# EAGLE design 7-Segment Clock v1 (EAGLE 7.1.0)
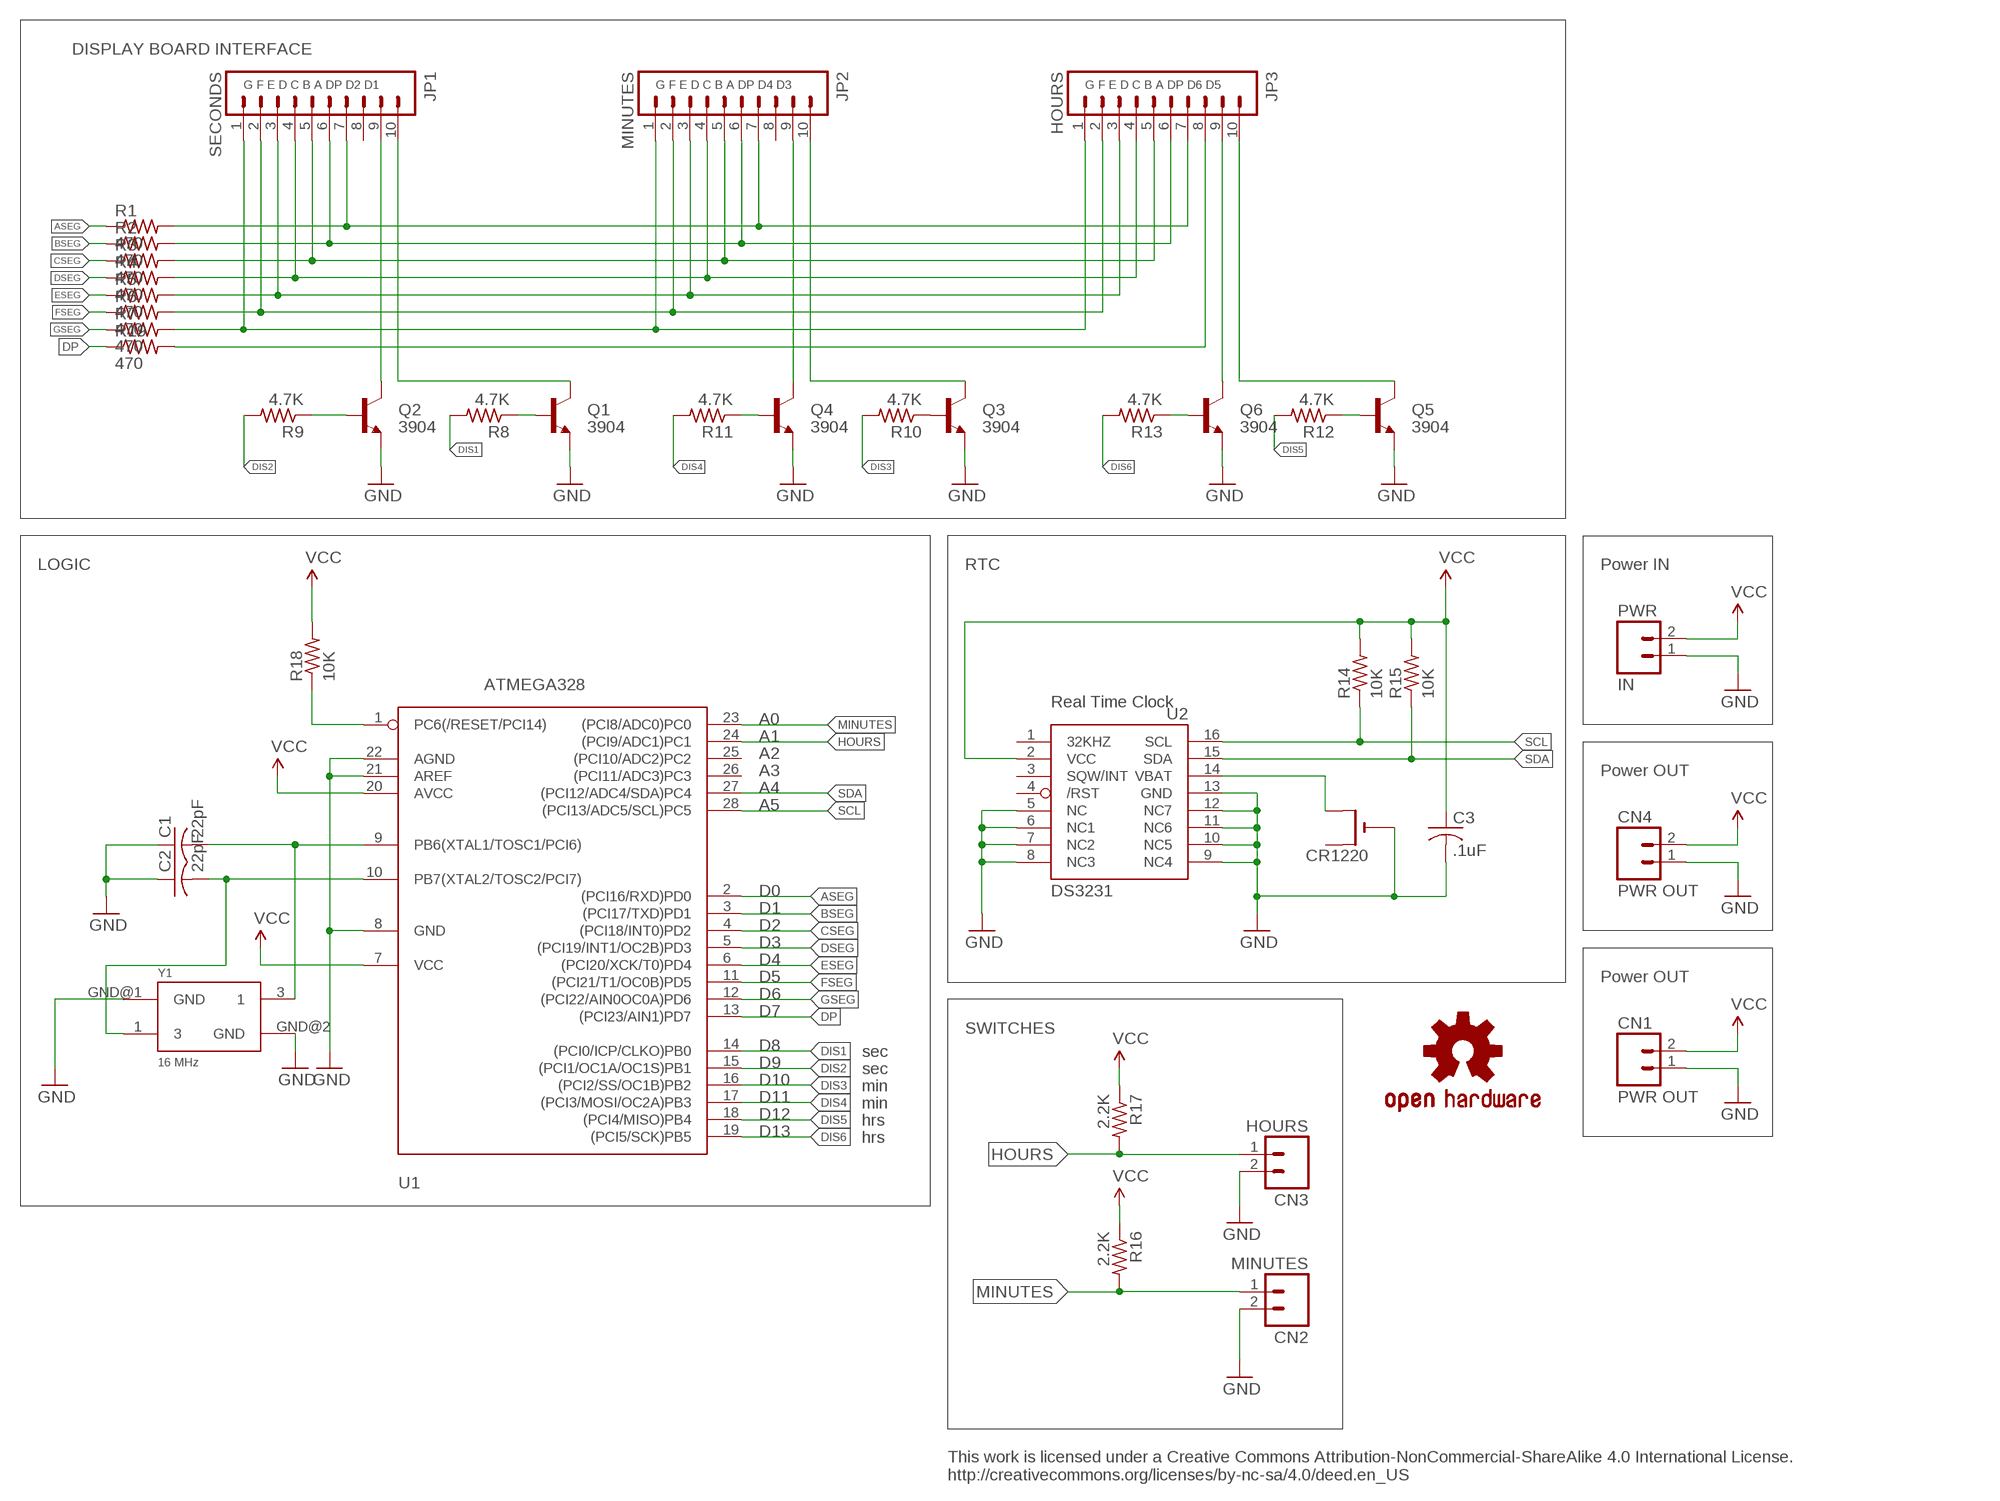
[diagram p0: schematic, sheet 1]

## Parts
C1  22pF  C-USC0805K  [C0805K]
C2  22pF  C-USC0805K  [C0805K]
C3  .1uF  C-USC0805K  [C0805K]
CN1  PWR OUT  M02PTH  [1X02]
CN2  MINUTES  M02PTH  [1X02]
CN3  HOURS  M02PTH  [1X02]
CN4  PWR OUT  M02PTH  [1X02]
CR1220  CR1220THM  [CR1220-THM]
JP1  SECONDS  M10NO_SILK  [1X10_NO_SILK]
JP2  MINUTES  M10NO_SILK  [1X10_NO_SILK]
JP3  HOURS  M10NO_SILK  [1X10_NO_SILK]
PWR  IN  M02PTH  [1X02]
Q1  3904  TRANSISTOR_NPNMMBT2222A  [SOT23]
Q2  3904  TRANSISTOR_NPNMMBT2222A  [SOT23]
Q3  3904  TRANSISTOR_NPNMMBT2222A  [SOT23]
Q4  3904  TRANSISTOR_NPNMMBT2222A  [SOT23]
Q5  3904  TRANSISTOR_NPNMMBT2222A  [SOT23]
Q6  3904  TRANSISTOR_NPNMMBT2222A  [SOT23]
R1  470  R-US_R0805  [R0805]
R2  470  R-US_R0805  [R0805]
R3  470  R-US_R0805  [R0805]
R4  470  R-US_R0805  [R0805]
R5  470  R-US_R0805  [R0805]
R6  470  R-US_R0805  [R0805]
R7  470  R-US_R0805  [R0805]
R8  4.7K  R-US_R0805  [R0805]
R9  4.7K  R-US_R0805  [R0805]
R10  4.7K  R-US_R0805  [R0805]
R11  4.7K  R-US_R0805  [R0805]
R12  4.7K  R-US_R0805  [R0805]
R13  4.7K  R-US_R0805  [R0805]
R14  10K  R-US_R0805  [R0805]
R15  10K  R-US_R0805  [R0805]
R16  2.2K  R-US_R0805  [R0805]
R17  2.2K  R-US_R0805  [R0805]
R18  10K  R-US_R0805  [R0805]
R19  470  R-US_R0805  [R0805]
U1  ATMEGA328  ATMEGA168PROUND  [DIL28-3-ROUND]
U2  DS3231  DS3231/SO  [SO16W]
U$7  OSHW-LOGOS  [OSHW-LOGO-S]
Y1  16 MHz  OSCILLATOR5X3  [CRYSTAL-SMD-5X3]

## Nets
ASEG: R1.1 U1.2((PCI16/RXD)PD0)
BSEG: R2.1 U1.3((PCI17/TXD)PD1)
CSEG: R3.1 U1.4((PCI18/INT0)PD2)
DIS1: R8.2 U1.14((PCI0/ICP/CLKO)PB0)
DIS2: R9.2 U1.15((PCI1/OC1A/OC1S)PB1)
DIS3: R10.2 U1.16((PCI2/SS/OC1B)PB2)
DIS4: R11.2 U1.17((PCI3/MOSI/OC2A)PB3)
DIS5: R12.2 U1.18((PCI4/MISO)PB4)
DIS6: R13.2 U1.19((PCI5/SCK)PB5)
DP: R19.1 U1.13((PCI23/AIN1)PD7)
DSEG: R4.1 U1.5((PCI19/INT1/OC2B)PD3)
ESEG: R5.1 U1.6((PCI20/XCK/T0)PD4)
FSEG: R6.1 U1.11((PCI21/T1/OC0B)PD5)
GND: C1.1 C2.1 C3.2 CN1.1 CN2.2 CN3.2 CN4.1 CR1220.- PWR.1 Q1.2(E) Q2.2(E) Q3.2(E) Q4.2(E) Q5.2(E) Q6.2(E) U1.8(GND) U1.21(AREF) U1.22(AGND) U2.5(NC) U2.6(NC1) U2.7(NC2) U2.8(NC3) U2.9(NC4) U2.10(NC5) U2.11(NC6) U2.12(NC7) U2.13(GND) Y1.GND@1(GND) Y1.GND@2(GND)
GSEG: R7.1 U1.12((PCI22/AIN0OC0A)PD6)
HOURS: CN3.1 R17.2 U1.24((PCI9/ADC1)PC1)
MINUTES: CN2.1 R16.2 U1.23((PCI8/ADC0)PC0)
N$1: Q1.1(B) R8.1
N$2: CR1220.+2(+1) U2.14(VBAT)
N$3: Q2.1(B) R9.1
N$4: JP1.7 JP2.7 JP3.7 R1.2
N$5: JP1.6 JP2.6 JP3.6 R2.2
N$6: JP1.5 JP2.5 JP3.5 R3.2
N$7: JP1.4 JP2.4 JP3.4 R4.2
N$8: Q3.1(B) R10.1
N$9: JP1.2 JP2.2 JP3.2 R6.2
N$10: JP1.1 JP2.1 JP3.1 R7.2
N$11: JP3.8 R19.2
N$12: JP1.9 Q2.3(C)
N$13: JP1.10 Q1.3(C)
N$14: JP2.9 Q4.3(C)
N$15: Q4.1(B) R11.1
N$16: Q5.1(B) R12.1
N$17: Q6.1(B) R13.1
N$18: JP2.10 Q3.3(C)
N$19: JP3.9 Q6.3(C)
N$20: JP3.10 Q5.3(C)
N$24: JP1.3 JP2.3 JP3.3 R5.2
N$36: R18.1 U1.1(PC6(/RESET/PCI14))
N$37: C1.2 U1.9(PB6(XTAL1/TOSC1/PCI6)) Y1.3
N$38: C2.2 U1.10(PB7(XTAL2/TOSC2/PCI7)) Y1.1
SCL: R14.1 U1.28((PCI13/ADC5/SCL)PC5) U2.16(SCL)
SDA: R15.1 U1.27((PCI12/ADC4/SDA)PC4) U2.15(SDA)
VCC: C3.1 CN1.2 CN4.2 PWR.2 R14.2 R15.2 R16.1 R17.1 R18.2 U1.7(VCC) U1.20(AVCC) U2.2(VCC)
Unconnected: CR1220.+1(+) JP1.8 JP2.8 U1.25((PCI10/ADC2)PC2) U1.26((PCI11/ADC3)PC3) U2.1(32KHZ) U2.3(SQW/INT) U2.4(/RST)

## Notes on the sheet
- DISPLAY BOARD INTERFACE
- G F E D C B A DP D2 D1 | G F E D C B A DP D4 D3 | G F E D C B A DP D6 D5
- LOGIC | RTC | Power IN
- Real Time Clock
- A0
- A1
- A2
- A3 | Power OUT
- A4
- A5
- D0
- D1
- D2
- D3
- D4
- D5 | Power OUT
- D6
- D7
- SWITCHES
- D8 | sec
- D9 | sec
- D10 | min
- D11 | min
- D12 | hrs
- D13 | hrs
- This work is licensed under a Creative Commons Attribution-NonCommercial-ShareAlike 4.0 International License.
  http://creativecommons.org/licenses/by-nc-sa/4.0/deed.en_US

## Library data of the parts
C1-C3 = adafruit:C-US: CAPACITOR, American symbol
CN1-CN4 PWR = SparkFun w:epaper:M02: Header 2
CR1220 = adafruit:CR1220: CR1216/CR1220/CR1225 12mm 3V lithium coin cell Great for battery packup. Both SMT and THM holders. Note the THM package has the ground pads on both sides of the PCB so that the masks are the same - this reduces the cost
JP1-JP3 = SparkFun-Connectors:M10: Header 10 Standard 10-pin 0.1" header. Use with straight break away headers (SKU : PRT-00116), right angle break away headers (PRT-00553), swiss pins (PRT-00743), machine pins (PRT-00117), and female headers (PRT-00115).
Q1-Q6 = SparkFun-DiscreteSemi:TRANSISTOR_NPN: Generic NPN BJT MMBT2222A - TRANS-08049 (SOT-23, 1A 40V) MPSA42 - TRANS-09116 (SOT-23, 500mA 300V) MMBT5088LT1G - TRANS-11160 (SOT-23, 50 mA 30V); PROD_ID: TRANS-08049; VALUE: MMBT2222A
R1-R19 = adafruit:R-US_: RESISTOR, American symbol
U1 = adafruit:ATMEGA168*P: MICROCONTROLLER 16 kBytes FLASH 1 kBytes SRAM 512 Bytes EEPROM USART 8-channel 10 bit ADC
U2 = adafruit:DS3231
U$7 = SparkFun:OSHW-LOGO: Open Source Hardware Logo This logo indicates the piece of hardware it is found on incorporates a OSHW license and/or adheres to the definition of open source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
Y1 = SparkFun-FreqCtrl:OSCILLATOR: Generic 5x3 and 7x5 oscillators

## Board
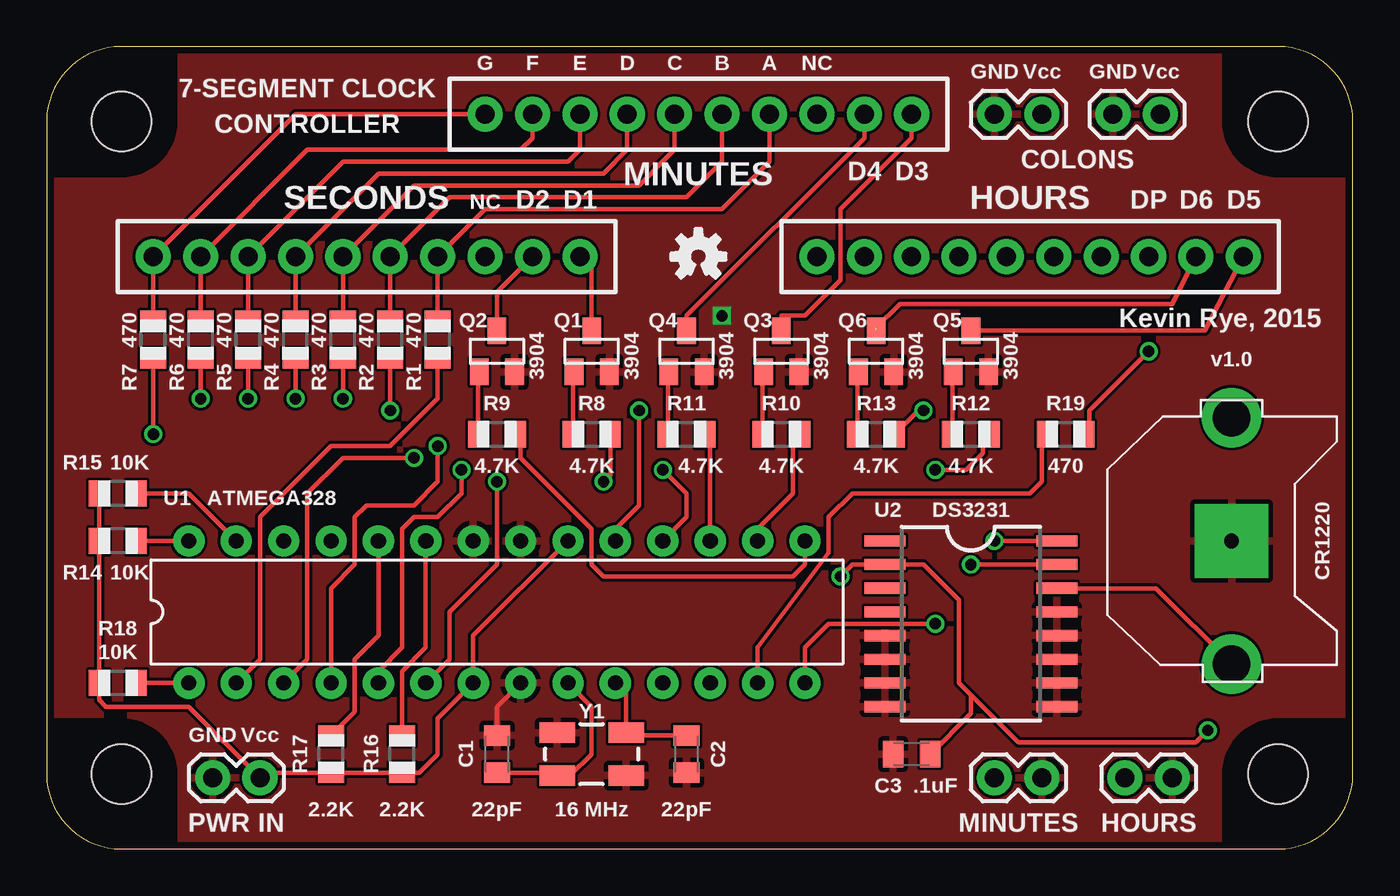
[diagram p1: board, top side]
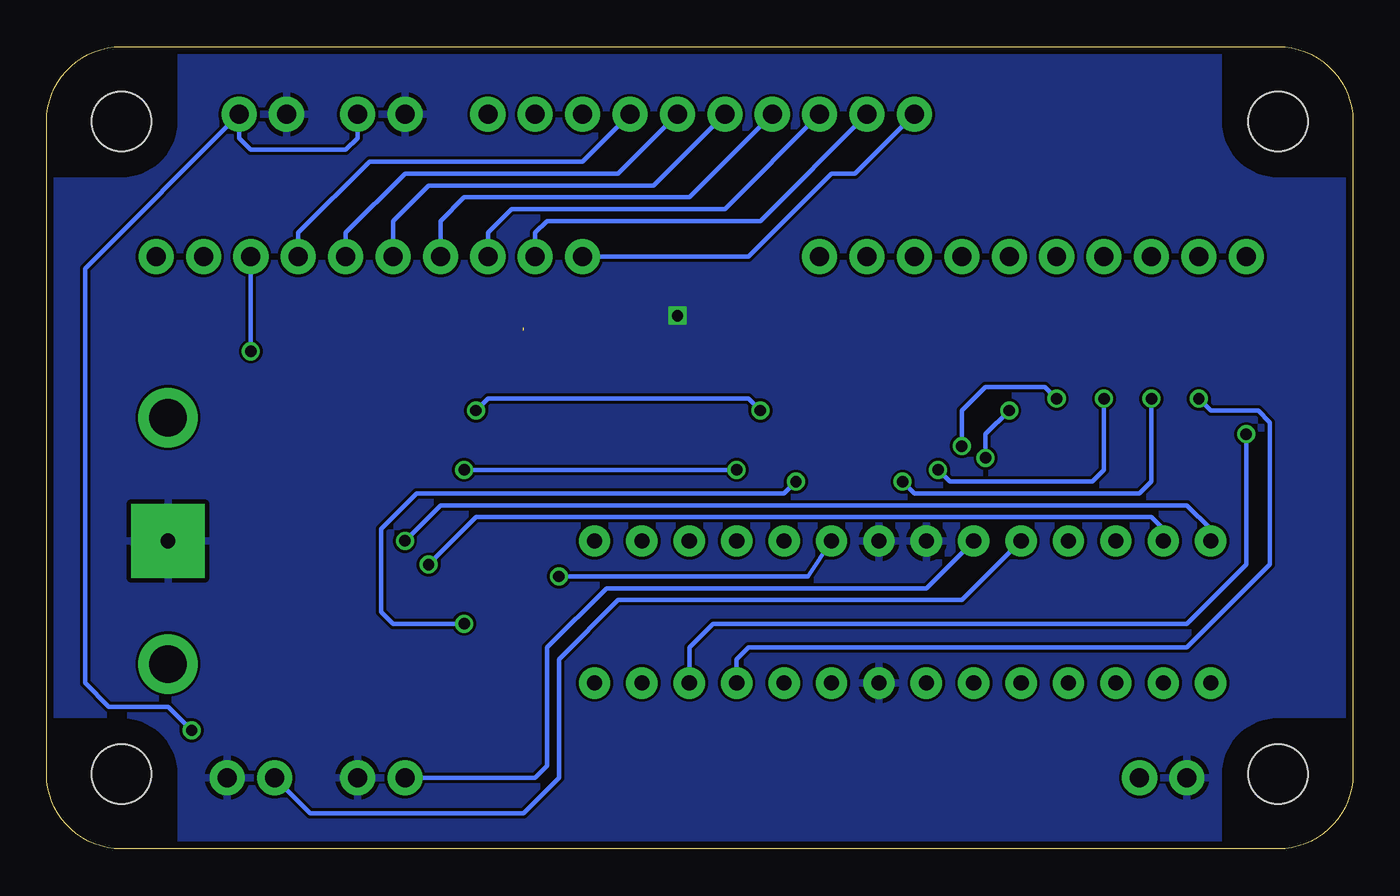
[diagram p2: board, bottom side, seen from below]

Size 70 x 43 mm. Coordinates in mm from the lower left corner, seen from the top.
Copper layers (1*16): Top 0.0356mm / dielectric 1.5011mm / Bottom 0.0356mm
Design rules "LaenPCBOrder": minimum track width 6mil, minimum drill 13mil, track to track 6mil, track to pad 6mil, pad to pad 6mil, via to via 6mil, smd to smd 6mil, copper to edge 15mil, drill to drill 6mil, minimum pad ring 7mil, minimum via ring 7mil, stop-mask expansion 3mil, vias tented up to drill 0mil, thermal gap 10mil

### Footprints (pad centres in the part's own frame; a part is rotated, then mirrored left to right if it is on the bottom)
C0805K = smd 1.1 x 1.4: 1 -1,0; 2 1,0
1X02 = drill 1.016 pad 1.88: 1 0,0; 2 2.54,0
CR1220-THM = drill 2 pad 3.175: +1 -6.604,0; +2 6.604,0 | drill 0.8 pad 3.962 square: - 0,0
1X10_NO_SILK = drill 1.016 pad 1.88: 1 0,0; 2 2.54,0; 3 5.08,0; 4 7.62,0; 5 10.16,0; 6 12.7,0; 7 15.24,0; 8 17.78,0; 9 20.32,0; 10 22.86,0
SOT23 = smd 1 x 1.4: 1 -0.95,-1.1; 2 0.95,-1.1; 3 0,1.1
R0805 = smd 1.1 x 1.4: 1 -1,0; 2 1,0
DIL28-3-ROUND = drill 0.813 pad 1.676: 1 -16.51,-3.81; 2 -13.97,-3.81; 3 -11.43,-3.81; 4 -8.89,-3.81; 5 -6.35,-3.81; 6 -3.81,-3.81; 7 -1.27,-3.81; 8 1.27,-3.81; 9 3.81,-3.81; 10 6.35,-3.81; 11 8.89,-3.81; 12 11.43,-3.81; 13 13.97,-3.81; 14 16.51,-3.81; 15 16.51,3.81; 16 13.97,3.81; 17 11.43,3.81; 18 8.89,3.81; 19 6.35,3.81; 20 3.81,3.81; 21 1.27,3.81; 22 -1.27,3.81; 23 -3.81,3.81; 24 -6.35,3.81; 25 -8.89,3.81; 26 -11.43,3.81; 27 -13.97,3.81; 28 -16.51,3.81
SO16W = smd 0.6 x 2.2: 1 -4.445,-4.6; 2 -3.175,-4.6; 3 -1.905,-4.6; 4 -0.635,-4.6; 5 0.635,-4.6; 6 1.905,-4.6; 7 3.175,-4.6; 8 4.445,-4.6; 9 4.445,4.6; 10 3.175,4.6; 11 1.905,4.6; 12 0.635,4.6; 13 -0.635,4.6; 14 -1.905,4.6; 15 -3.175,4.6; 16 -4.445,4.6
DP7043_V1 = hole 3.2: 4,4; 66,4; 66,39; 4,39
CRYSTAL-SMD-5X3 = smd 1.9 x 1.1: 1 -1.85,-1.15; 3 1.85,1.15; GND@1 -1.85,1.15; GND@2 1.85,-1.15

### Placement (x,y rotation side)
C1  24.13,5.08 270 top
C2  34.29,5.08 90 top
C3  46.35,5.08 180 top
CN1  50.8,39.37 0 top
CN2  50.8,3.81 0 top
CN3  57.78,3.81 0 top
CN4  57.15,39.37 0 top
CR1220  63.5,16.51 270 top
JP1  5.71,31.75 0 top
JP2  23.5,39.37 0 top
JP3  41.27,31.75 0 top
PWR  8.89,3.81 0 top
Q1  29.21,26.67 0 top
Q2  24.13,26.67 0 top
Q3  39.37,26.67 0 top
Q4  34.29,26.67 0 top
Q5  49.53,26.67 0 top
Q6  44.45,26.67 0 top
R1  20.95,27.31 90 top
R2  18.41,27.31 90 top
R3  15.88,27.31 90 top
R4  13.34,27.31 90 top
R5  10.79,27.31 90 top
R6  8.26,27.31 90 top
R7  5.71,27.31 90 top
R8  29.21,22.22 0 top
R9  24.13,22.22 0 top
R10  39.37,22.22 0 top
R11  34.29,22.22 0 top
R12  49.53,22.22 0 top
R13  44.45,22.22 0 top
R14  3.81,16.51 180 top
R15  3.81,19.05 180 top
R16  19.05,5.08 90 top
R17  15.24,5.08 90 top
R18  3.81,8.89 180 top
R19  54.61,22.22 0 top
U1  24.13,12.7 0 top
U2  49.53,12.07 270 top
U$2  [DP7043_V1]  0,0 0 top
U$7  34.92,31.75 0 top
Y1  29.21,5.08 180 top

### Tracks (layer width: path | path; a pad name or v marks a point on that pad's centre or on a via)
ASEG
  Top 0.254: U1.2 11.43,10.16 11.43,17.78 15.24,21.59 18.41,21.59 20.95,24.13 R1.1 20.95,24.77
BSEG  (via drill 0.61)
  Top 0.254: U1.3 13.97,10.16 13.97,19.05 15.88,20.96 v19.68,20.96 | v18.41,23.5 R2.1
  Bottom 0.254: v19.68,20.96 19.68,22.22 v18.41,23.5
CSEG  (via drill 0.61)
  Top 0.254: U1.4 15.24,13.97 16.51,15.24 16.51,17.78 17.14,18.41 19.68,18.41 20.95,19.68 v20.95,21.59 | v15.88,24.13 R3.1
  Bottom 0.254: v20.95,21.59 20.95,23.5 19.68,24.77 16.51,24.77 v15.88,24.13
DIS1  (via drill 0.61)
  Top 0.254: R8.2 30.21,20.05 v29.84,19.68 | v47.62,12.07 41.91,12.07 40.64,10.8 U1.14
  Bottom 0.254: v29.84,19.68 30.48,19.05 50.16,19.05 52.07,17.14 52.07,12.7 51.44,12.07 v47.62,12.07
DIS2
  Top 0.254: U1.15 40.64,15.24 40.01,14.61 29.84,14.61 29.21,15.24 29.21,17.14 25.4,20.96 25.4,21.96 R9.2
DIS3
  Top 0.254: U1.16 38.1,17.14 40.01,19.05 40.01,21.86 R10.2
DIS4
  Top 0.254: U1.17 35.56,21.96 R11.2
DIS5  (via drill 0.61)
  Top 0.254: v47.62,20.32 49.27,20.32 50.16,21.22 50.16,21.86 R12.2 | v33.02,20.32 34.29,19.05 34.29,17.78 U1.18
  Bottom 0.254: v33.02,20.32 v47.62,20.32
DIS6  (via drill 0.61)
  Top 0.254: U1.19 30.48,17.14 31.75,18.41 v31.75,23.5 | v46.99,23.5 46.72,23.5 R13.2
  Bottom 0.254: v31.75,23.5 32.38,24.13 46.35,24.13 v46.99,23.5
DP
  Top 0.254: U1.13 38.1,10.8 41.91,15.88 41.91,17.78 43.18,19.05 52.7,19.05 53.34,19.68 53.34,21.96 R19.1
DSEG  (via drill 0.61)
  Top 0.254: U1.5 17.78,9.53 19.05,10.8 19.05,17.14 19.68,17.78 20.95,17.78 22.23,19.05 v22.23,20.32 | R4.1 v13.34,24.13
  Bottom 0.254: v13.34,24.13 13.34,20.32 13.97,19.68 21.59,19.68 v22.23,20.32
ESEG  (via drill 0.61)
  Top 0.254: U1.6 21.59,10.16 21.59,12.7 24.13,15.24 v24.13,19.68 | v10.79,24.13 R5.1
  Bottom 0.254: v24.13,19.68 23.5,19.05 11.43,19.05 10.79,19.68 v10.79,24.13
FSEG  (via drill 0.61)
  Top 0.254: v8.26,24.13 R6.1
  Bottom 0.254: U1.11 33.02,10.16 32.38,10.8 8.89,10.8 4.45,15.24 4.45,22.86 5.08,23.5 7.62,23.5 v8.26,24.13
GND  (via drill 0.61)
  Top 0.254: C1.1 24.13,7.62 U1.8
  other vias: 36.2,28.57
  pour Top: -1.27,44.45 71.75,44.45 71.75,-1.27 -1.27,-1.27
  pour Bottom: -0.64,43.81 71.12,43.81 71.12,-0.63 -0.64,-0.63
GSEG  (via drill 0.61)
  Top 0.254: v5.71,22.22 R7.1
  Bottom 0.254: U1.12 35.56,10.8 34.29,12.07 8.89,12.07 5.71,15.24 v5.71,22.22
HOURS
  Top 0.254: 15.24,6.35 R17.2 16.51,7.35 16.51,10.16 17.78,11.43 U1.24
  Bottom 0.254: CN3.1 55.88,1.91 44.45,1.91 42.55,3.81 42.55,10.16 39.37,13.34 20.95,13.34 U1.24
MINUTES
  Top 0.254: R16.2 19.05,9.53 20.32,10.8 U1.23
  Bottom 0.254: CN2.1 43.81,3.81 43.18,4.45 43.18,10.8 40.01,13.97 22.86,13.97 U1.23
N$1
  Top 0.254: R8.1 28.21,25.52 Q1.1
N$2
  Top 0.254: U2.14 59.44,13.97 CR1220.+2
N$3
  Top 0.254: R9.1 23.13,25.52 Q2.1
N$4
  Top 0.254: R1.2 JP1.7 23.5,34.29 36.2,34.29 38.73,36.83 JP2.7
  Bottom 0.254: JP3.7 56.52,33.02 52.7,36.83 41.27,36.83 JP2.7
N$5
  Top 0.254: R2.2 JP1.6 21.59,34.92 34.29,34.92 36.2,36.83 JP2.6
  Bottom 0.254: JP3.6 53.98,33.02 50.8,36.2 39.37,36.2 JP2.6
N$6
  Top 0.254: R3.2 JP1.5 19.68,35.56 31.75,35.56 33.66,37.47 JP2.5
  Bottom 0.254: JP2.5 37.47,35.56 49.53,35.56 51.44,33.66 JP3.5
N$7
  Top 0.254: R4.2 JP1.4 17.78,36.2 29.84,36.2 31.11,37.47 JP2.4
  Bottom 0.254: JP3.4 48.9,33.66 47.62,34.92 35.56,34.92 JP2.4
N$8
  Top 0.254: R10.1 38.37,25.52 Q3.1
N$9
  Top 0.254: R6.2 JP1.2 13.97,37.47 25.4,37.47 26.04,38.1 JP2.2
  Bottom 0.254: JP3.2 43.81,33.02 43.18,33.66 31.75,33.66 JP2.2
N$10
  Top 0.254: R7.2 JP1.1 13.34,39.37 JP2.1
  Bottom 0.254: JP3.1 32.38,31.75 27.94,36.2 26.67,36.2 JP2.1
N$11  (via drill 0.61)
  Top 0.254: v59.05,26.67 55.88,23.5 55.88,22.5 R19.2
  Bottom 0.254: v59.05,26.67 JP3.8
N$12
  Top 0.254: Q2.3 24.13,29.85 JP1.9
N$13
  Top 0.254: Q1.3 29.21,31.11 JP1.10
N$14
  Top 0.254: Q4.3 34.29,28.57 43.81,38.1 JP2.9
N$15
  Top 0.254: R11.1 33.29,25.52 Q4.1
N$16
  Top 0.254: R12.1 48.53,25.52 Q5.1
N$17
  Top 0.254: R13.1 43.45,25.52 Q6.1
N$18
  Top 0.254: Q3.3 39.37,28.57 40.64,28.57 42.55,30.48 42.55,34.29 46.35,38.1 JP2.10
N$19  (1 unrouted)
  Top 0.254: 44.45,27.94 45.72,29.21 60.33,29.21 JP3.9
N$20
  Top 0.254: Q5.3 62.06,27.77 JP3.10
N$24
  Top 0.254: R5.2 JP1.3 15.88,36.83 27.94,36.83 28.57,37.47 JP2.3
  Bottom 0.254: JP3.3 46.35,33.02 45.09,34.29 33.66,34.29 JP2.3
N$36
  Top 0.254: R18.1 U1.1
N$37
  Top 0.254: U1.9 29.21,7.62 29.21,5.08 28.06,3.93 Y1.3 27.21,4.08 C1.2
N$38
  Top 0.254: U1.10 31.06,8.31 Y1.1 31.21,6.08 C2.2
SCL  (via drill 0.61)
  Top 0.254: v50.8,16.51 U2.16 | R14.1 U1.28
  Bottom 0.254: U1.28 7.62,17.14 8.89,18.41 48.9,18.41 v50.8,16.51
SDA  (via drill 0.61)
  Top 0.254: v49.53,15.24 U2.15 | U1.27 7.62,19.05 R15.1
  Bottom 0.254: U1.27 10.16,17.14 10.79,17.78 46.99,17.78 v49.53,15.24
VCC  (via drill 0.61)
  Top 0.254: U2.2 46.99,15.24 48.9,13.34 48.9,8.89 49.53,8.25 | U1.20 22.86,11.43 U1.7 20.95,6.98 20.95,5.08 19.95,4.08 R16.1 R17.1 11.7,4.08 PWR.2 7.62,7.62 3.17,7.62 2.81,7.98 R18.2 R14.2 R15.2 | 49.53,8.25 52.07,5.71 61.59,5.71 v62.23,6.35 | v42.55,14.61 43.18,15.24 U2.2 | 45.09,15.24 U2.2 | C3.1 49.53,7.25 49.53,8.25
  Bottom 0.254: U1.20 29.21,14.61 v42.55,14.61 | v62.23,6.35 63.5,7.62 66.67,7.62 67.94,8.89 67.94,31.11 CN4.2 59.69,38.1 59.05,37.47 53.98,37.47 53.34,38.1 CN1.2

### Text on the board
Unrouted: This work is licensed under a Creative Commons Attribution-NonCommercial-ShareAlike 4.0 International License. / http://creativecommons.org/licenses/by-nc-sa/4.0/deed.en_US
tPlace: G | F | E | D | C | B | A | NC | 7-SEGMENT CLOCK | GND | Vcc | GND | Vcc | CONTROLLER | D4 | D3 | COLONS | NC | D2 | D1 | DP | D6 | D5 | Kevin Rye, 2015 | v1.0 | GND | Vcc | PWR IN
